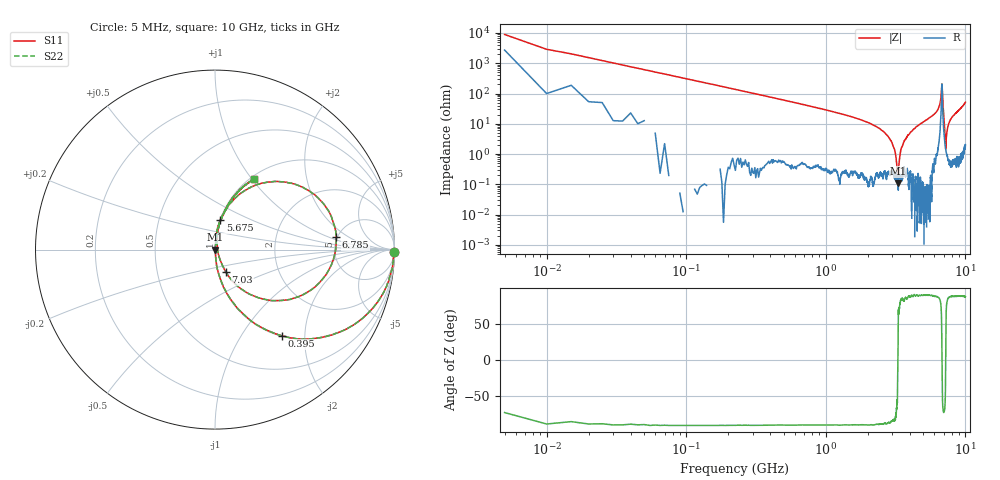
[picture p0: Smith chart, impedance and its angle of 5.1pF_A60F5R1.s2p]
! Amotech Co.,Ltd.
! http://www.amotech.co.kr/
! Part Number: A60F5R1
! These Parameters are Measured in Series Mode Connection
! Operation Temp=25[degC], DC Bias Voltage=0[V]
! Freq. Start=5[MHz] Stop=10[GHz], 2000[Steps]
! Date: Monday, July 20, 2020, 04:03:02
# GHZ S RI R 50.000000
!Freq.(Hz) S11(Real) S11(Imag) S21(Real) S21(Imag) S12(Real) S12(Imag) S22(Real) S22(Imag)
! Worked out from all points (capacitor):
!   2000 points, 5 MHz to 10 GHz, reference 50 ohm
!   read as one part in series: C = 5.17 pF near 55 MHz
!   lowest |Z| = 107 mohm at 3.29 GHz (marker M1)
!   series resonance near 3.288 GHz, so ESL is about 450 pH
!   S11 on the Smith chart (normalised r, x): 5 MHz: open; 395 MHz: 1.01, -1.54; 5.675 GHz: 1.00, +0.34; 6.785 GHz: 4.88, +1.28; 7.03 GHz: 1.09, -0.28; 10 GHz: 1.04, +1.03
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0.005  0.9965 -0.0106  0.00352 0.0106  0.00352 0.0106  0.9965 -0.0106
0.065  0.9572 -0.2021  0.0428 0.2021  0.0428 0.2021  0.9572 -0.2021
0.115  0.8782 -0.327  0.1218 0.327  0.1218 0.327  0.8782 -0.327
0.395  0.3738 -0.4807  0.6262 0.4807  0.6262 0.4807  0.3738 -0.4807
1.675  0.0238 -0.1452  0.9762 0.1452  0.9762 0.1452  0.0238 -0.1452
2.92  0.00314 -0.0279  0.9969 0.0279  0.9969 0.0279  0.00314 -0.0279
3.13  0.00156 -0.0122  0.9984 0.0122  0.9984 0.0122  0.00156 -0.0122
3.29  0.00107 7.72e-05  0.9989 -7.72e-05  0.9989 -7.72e-05  0.00107 7.72e-05
3.34  0.00182 0.00428  0.9982 -0.00428  0.9982 -0.00428  0.00182 0.00428
3.45  0.0018 0.0136  0.9982 -0.0136  0.9982 -0.0136  0.0018 0.0136
3.665  0.0036 0.0277  0.9964 -0.0277  0.9964 -0.0277  0.0036 0.0277
5.005  0.0139 0.1151  0.9861 -0.1151  0.9861 -0.1151  0.0139 0.1151
5.675  0.0298 0.1661  0.9702 -0.1661  0.9702 -0.1661  0.0298 0.1661
6.42  0.1096 0.2841  0.8904 -0.2841  0.8904 -0.2841  0.1096 0.2841
6.67  0.3586 0.3789  0.6414 -0.3789  0.6414 -0.3789  0.3586 0.3789
6.785  0.6753 0.0709  0.3247 -0.0709  0.3247 -0.0709  0.6753 0.0709
6.88  0.3508 -0.2843  0.6492 0.2843  0.6492 0.2843  0.3508 -0.2843
7.03  0.0613 -0.1261  0.9387 0.1261  0.9387 0.1261  0.0613 -0.1261
7.23  0.014 0.00452  0.986 -0.00452  0.986 -0.00452  0.014 0.00452
7.525  0.0136 0.0857  0.9864 -0.0857  0.9864 -0.0857  0.0136 0.0857
8.335  0.0447 0.1914  0.9553 -0.1914  0.9553 -0.1914  0.0447 0.1914
10  0.2191 0.3944  0.7809 -0.3944  0.7809 -0.3944  0.2191 0.3944
